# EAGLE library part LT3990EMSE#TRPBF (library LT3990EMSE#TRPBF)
Switching Voltage Regulators 60V, 350mA Step-Down Regulator with 2uA Quiescent Current and Integrated Diodes in MS16E Source: Datasheet
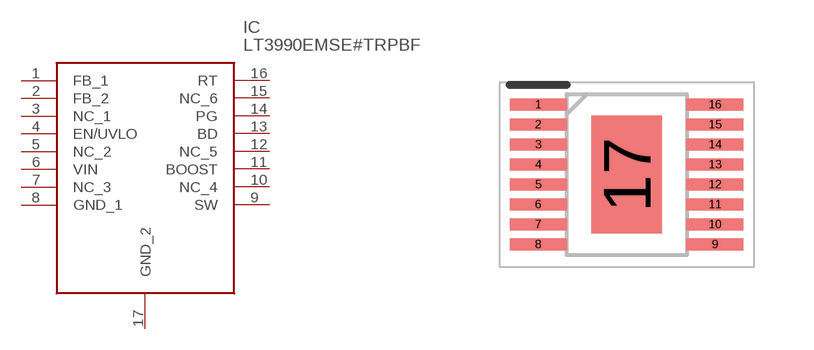
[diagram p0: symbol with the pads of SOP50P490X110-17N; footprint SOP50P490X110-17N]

Designator prefix IC

## LT3990EMSE#TRPBF (Description: Switching Voltage Regulators 60V, 350mA Step-Down Regulator with 2uA Quiescent Current and Integrated Diodes in MS16E; Height: 1.1mm; Manufacturer_Name: Analog Devices; Manufacturer_Part_Number: LT3990EMSE#TRPBF; Mouser_Part_Number: 584-LT3990EMSE#TRPBF; Mouser_Price-Stock: https://www.mouser.co.uk/ProductDetail/Analog-Devices/LT3990EMSETRPBF?qs=hVkxg5c3xu84JUDF%2FgczpA%3D%3D)  [SOP50P490X110-17N]
1  FB_1
2  FB_2
3  NC_1
4  EN/UVLO
5  NC_2
6  VIN
7  NC_3
8  GND_1
9  SW
10  NC_4
11  BOOST
12  NC_5
13  BD
14  PG
15  NC_6
16  RT
17  GND_2

## Footprint SOP50P490X110-17N (pad centres in mm)
MSE Package 16-Lead Plastic MSOP, Exposed Die Pad
smd 1.425 x 0.3: 1 -2.212,1.75; 2 -2.212,1.25; 3 -2.212,0.75; 4 -2.212,0.25; 5 -2.212,-0.25; 6 -2.212,-0.75; 7 -2.212,-1.25; 8 -2.212,-1.75; 9 2.212,-1.75; 10 2.212,-1.25; 11 2.212,-0.75; 12 2.212,-0.25; 13 2.212,0.25; 14 2.212,0.75; 15 2.212,1.25; 16 2.212,1.75
smd 1.753 x 2.947: 17 0,0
